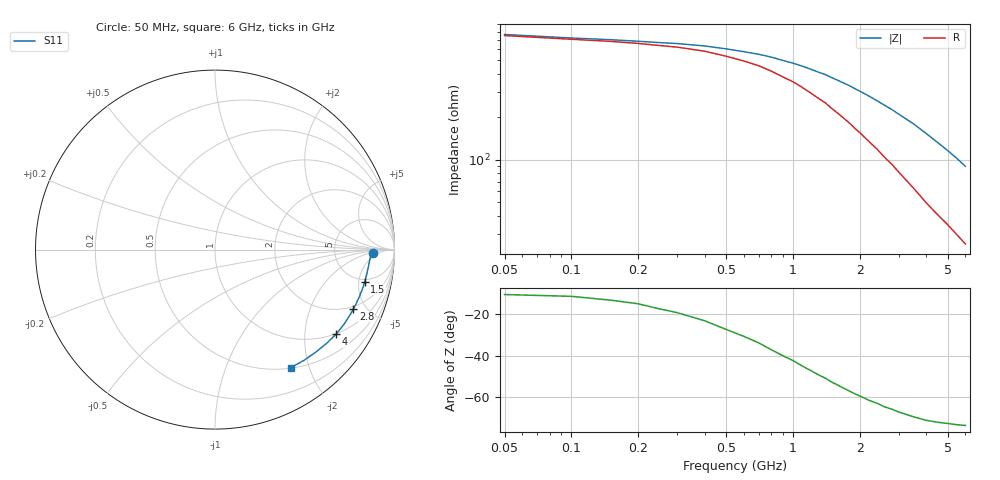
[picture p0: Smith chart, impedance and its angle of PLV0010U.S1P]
! Infineon Technologies  Discrete & RF Semiconductors
! BAR 64-04W /-05W /-06W
! Si PIN Diode in SOT323
! IF = 0.01 mA
! S-Parameters:  October  2008
# GHz  S  MA  R  50
!  f  S11
! GHz  MAG  ANG
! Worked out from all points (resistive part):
!   34 points, 50 MHz to 6 GHz, reference 50 ohm
!   read as one part to ground: R = 749 ohm at 50 MHz
!   S11 on the Smith chart (normalised r, x): 50 MHz: 15, -3; 1.5 GHz: 4.57, -6.02; 2.8 GHz: 1.85, -4.10; 4 GHz: 0.99, -2.88; 6 GHz: 0.51, -1.72
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0.05  0.8789 -1.4
0.1  0.8726 -1.6
0.2  0.868 -2.2
0.25  0.8669 -2.6
0.4  0.8647 -3.6
0.5  0.8632 -4.4
0.7  0.8606 -5.8
0.8  0.8601 -6.6
0.9  0.8584 -7.4
1  0.8574 -8.1
1.1  0.8569 -8.9
1.3  0.8547 -10.5
1.4  0.8541 -11.2
1.5  0.8533 -12.1
1.6  0.852 -12.9
1.8  0.8505 -14.5
1.9  0.8496 -15.4
2.2  0.8463 -17.9
2.4  0.843 -19.6
2.6  0.8418 -21.4
2.8  0.8386 -23.1
3  0.8368 -25.0
3.5  0.8312 -29.6
4  0.8231 -34.8
4.5  0.812 -40.1
5  0.8011 -45.4
5.5  0.7918 -51.1
6  0.7817 -57.2
